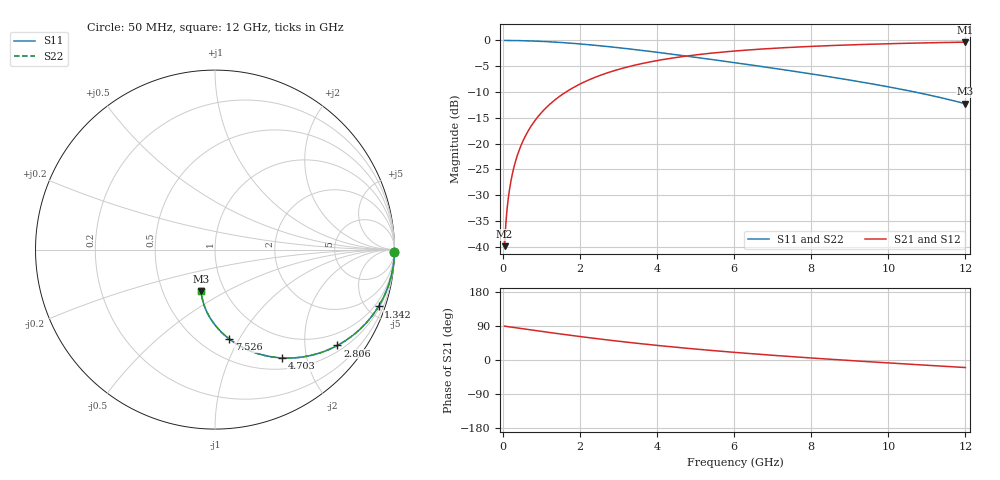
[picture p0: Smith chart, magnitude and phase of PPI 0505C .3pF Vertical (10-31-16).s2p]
# GHz S MA R 50
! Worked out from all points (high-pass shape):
!   1601 points, 50 MHz to 12 GHz, reference 50 ohm
!   highest |S21| = -0.33 dB at 12 GHz (marker M1); lowest = -39.9 dB at 50 MHz (marker M2)
!   |S21| within 3 dB of the highest: 4.478 GHz to end of sweep
!   lowest |S11| = -12.3 dB at 12 GHz (marker M3), VSWR 1.64, Z = 38.8 - j19 ohm
!   |S11| at or under -10 dB: 10.69 GHz to end of sweep
!   |S22| runs from -12.3 to 0.0 dB; largest |S21 - S12| = 0
!   S11 on the Smith chart (normalised r, x): 50 MHz: open; 1.342 GHz: 0.64, -5.86; 2.806 GHz: 0.65, -2.77; 4.703 GHz: 0.66, -1.60; 7.526 GHz: 0.68, -0.91; 12 GHz: 0.78, -0.38
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0.05  0.9999 -0.7  0.01012 89.3  0.01012 89.3  0.9999 -0.7
0.079875  0.9999 -1.2  0.01617 88.8  0.01617 88.8  0.9999 -1.2
0.1470937  0.9995 -2.1  0.02977 87.9  0.02977 87.9  0.9995 -2.1
0.2068437  0.9991 -3.0  0.04185 87.0  0.04185 87.0  0.9991 -3.0
0.3039375  0.9981 -4.4  0.06143 85.6  0.06143 85.6  0.9981 -4.4
0.4309062  0.9962 -6.2  0.08694 83.7  0.08694 83.7  0.9962 -6.2
0.5952188  0.9927 -8.6  0.1197 81.4  0.1197 81.4  0.9927 -8.6
0.8043438  0.9869 -11.6  0.1609 78.4  0.1609 78.4  0.9869 -11.6
1.050812  0.9779 -15.1  0.2084 74.9  0.2084 74.9  0.9779 -15.1
1.342094  0.9646 -19.2  0.2628 70.8  0.2628 70.8  0.9646 -19.2
1.670719  0.9466 -23.6  0.3214 66.3  0.3214 66.3  0.9466 -23.6
2.044156  0.9227 -28.6  0.3841 61.4  0.3841 61.4  0.9227 -28.6
2.805969  0.8663 -38.0  0.4978 51.9  0.4978 51.9  0.8663 -38.0
3.403469  0.8179 -44.9  0.5733 45.0  0.5733 45.0  0.8179 -44.9
4.038312  0.7652 -51.6  0.6414 38.2  0.6414 38.2  0.7652 -51.6
4.703031  0.7106 -58.2  0.7008 31.7  0.7008 31.7  0.7106 -58.2
6.025  0.6082 -69.7  0.7902 20.1  0.7902 20.1  0.6082 -69.7
7.526219  0.5043 -80.9  0.8592 8.6  0.8592 8.6  0.5043 -80.9
8.019156  0.4728 -84.3  0.8766 5.2  0.8766 5.2  0.4728 -84.3
8.990094  0.4136 -90.7  0.9054 -1.3  0.9054 -1.3  0.4136 -90.7
10.01331  0.3544 -97.0  0.9295 -7.8  0.9295 -7.8  0.3544 -97.0
12  0.2433 -108.5  0.9633 -19.9  0.9633 -19.9  0.2433 -108.5
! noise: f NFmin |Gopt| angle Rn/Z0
0.05  0.002885  0.9899  0.7078  0.06565
1.372  0.006151  0.8109  9.496  0.006734
2.701  0.009109  0.7346  13.32  0.006763
4.031  0.01181  0.6918  16.69  0.007311
5.36  0.01438  0.6639  19.97  0.007958
6.682  0.01687  0.6448  23.2  0.008647
8.012  0.01937  0.6315  26.41  0.009386
9.341  0.02192  0.6226  29.57  0.01018
10.67  0.02454  0.6174  32.67  0.01105
12  0.02728  0.6154  35.7  0.01202
